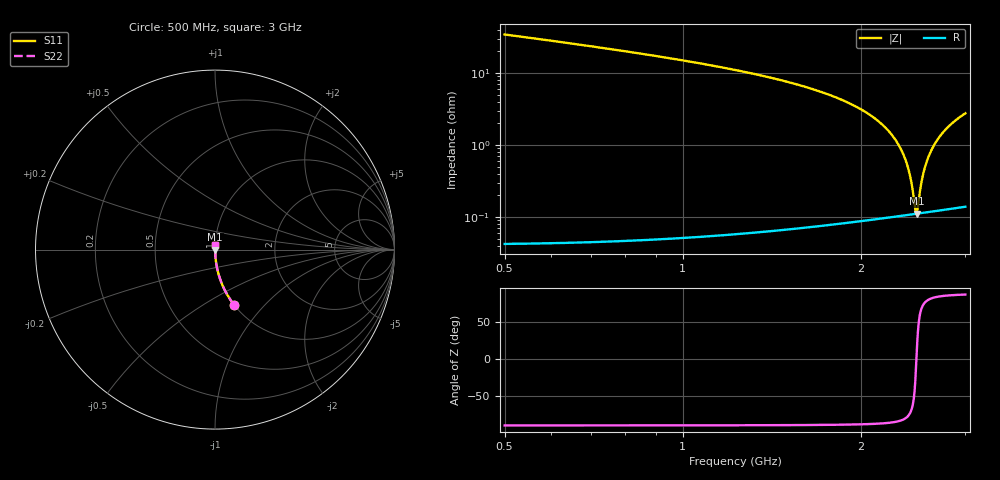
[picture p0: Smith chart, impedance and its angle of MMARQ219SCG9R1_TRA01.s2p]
! MMARQ219SCG9R1_TRA01  S-PARAMETER MODEL  ( General Type )
! Model Generated by TAIYO YUDEN Corporation (http://www.ty-top.com)
! Version 1.0
! TAIYO YUDEN Control No. 160201
! Copyright(c) 2016 TAIYO YUDEN CO.,LTD. All Rights Reserved.
! Product Description (link to TY-COMPAS)
! https://ds.yuden.co.jp/TYCOMPAS/or/detail?pn=MMARQ219SCG9R1CTRA01&u=M
! Products Name : Multilayer Ceramic Capacitors
! Characteristics :
!  Capacitance : 9.1 pF , Rated Voltage : 250V , TCC : CG / C0G
!  Case Size : 2.0 x 1.25 / 0.079 x 0.049 [mm/inch] , Thickness : 0.85 / 0.033 [mm/inch]
!  (Conditions: Temperature = 25 degC , DC Bias Current/Voltage = 0A / 0V)
! External Node Assignments :
!  1  o---| |---o  2
! GND o---------o GND
! Frequency Range : 500MHz  -  3000MHz  [ 401 STEP ]
# MHz S RI R 50
! Freq[MHz].  S11 Real  S11 Imag  S21 Real  S21 Imag  S12 Real  S12 Imag  S22 Real  S22 Imag
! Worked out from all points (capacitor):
!   401 points, 500 MHz to 3 GHz, reference 50 ohm
!   read as one part in series: C = 8.9 pF near 512.5 MHz
!   lowest |Z| = 111 mohm at 2.481 GHz (marker M1)
!   series resonance near 2.48 GHz, so ESL is about 460 pH
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500  0.1057 -0.3069  0.8943 0.3069  0.8943 0.3069  0.1057 -0.3069
918.75  0.0279 -0.1632  0.9721 0.1632  0.9721 0.1632  0.0279 -0.1632
1337.5  0.00949 -0.0938  0.9905 0.0938  0.9905 0.0938  0.00949 -0.0938
1750  0.00338 -0.051  0.9966 0.051  0.9966 0.051  0.00338 -0.051
1987.5  0.0019 -0.032  0.9981 0.032  0.9981 0.032  0.0019 -0.032
2168.75  0.00132 -0.0193  0.9987 0.0193  0.9987 0.0193  0.00132 -0.0193
2287.5  0.00114 -0.0116  0.9989 0.0116  0.9989 0.0116  0.00114 -0.0116
2368.75  0.00109 -0.00659  0.9989 0.00659  0.9989 0.00659  0.00109 -0.00659
2393.75  0.00109 -0.00508  0.9989 0.00508  0.9989 0.00508  0.00109 -0.00508
2418.75  0.00109 -0.00358  0.9989 0.00358  0.9989 0.00358  0.00109 -0.00358
2437.5  0.00109 -0.00247  0.9989 0.00247  0.9989 0.00247  0.00109 -0.00247
2468.75  0.0011 -0.000645  0.9989 0.000645  0.9989 0.000645  0.0011 -0.000645
2481.25  0.00111 7.99e-05  0.9989 -7.99e-05  0.9989 -7.99e-05  0.00111 7.99e-05
2493.75  0.00111 0.000801  0.9989 -0.000801  0.9989 -0.000801  0.00111 0.000801
2518.75  0.00113 0.00223  0.9989 -0.00223  0.9989 -0.00223  0.00113 0.00223
2537.5  0.00115 0.0033  0.9989 -0.0033  0.9989 -0.0033  0.00115 0.0033
2562.5  0.00117 0.0047  0.9988 -0.0047  0.9988 -0.0047  0.00117 0.0047
2587.5  0.0012 0.0061  0.9988 -0.0061  0.9988 -0.0061  0.0012 0.0061
2656.25  0.00129 0.00986  0.9987 -0.00986  0.9987 -0.00986  0.00129 0.00986
2743.75  0.00145 0.0145  0.9985 -0.0145  0.9985 -0.0145  0.00145 0.0145
2862.5  0.00173 0.0206  0.9983 -0.0206  0.9983 -0.0206  0.00173 0.0206
3000  0.00214 0.0274  0.9979 -0.0274  0.9979 -0.0274  0.00214 0.0274
